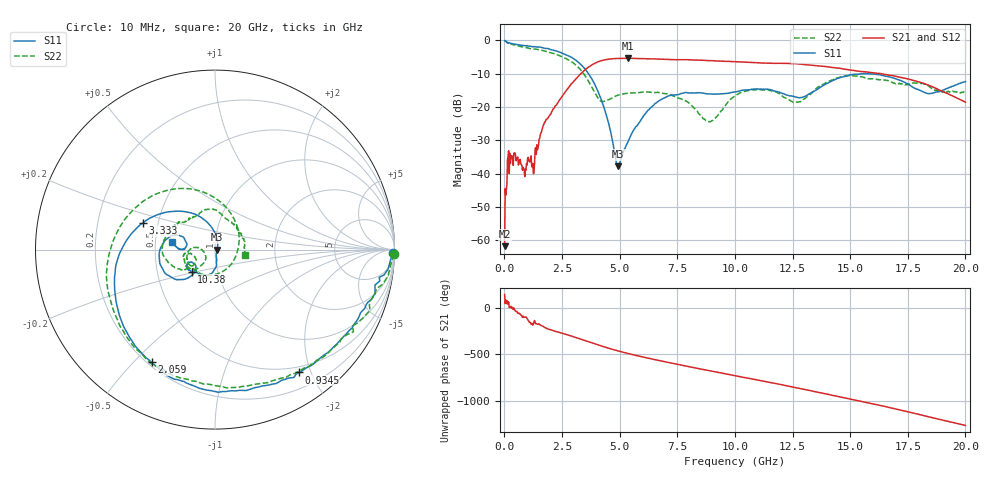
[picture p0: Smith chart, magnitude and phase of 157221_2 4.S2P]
!  2-Port S-parameters saved by WinCal
! VAR MeasName=S-Parameters (CALIBRATED_DATA) read from VNA (N5242A)
! VAR MeasDate=2015-5-26 16:47:30
! VAR NAME=157221_2 4
! VAR FILENAME=157221_2 4.S2P
! VAR DATE=2015-5-26 16:47:30
! VAR PHYS_PORTS=1,2
# Hz S DB R 50
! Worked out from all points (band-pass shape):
!   801 points, 10 MHz to 20 GHz, reference 50 ohm
!   highest |S21| = -5.38 dB at 5.357 GHz (marker M1); lowest = -61.8 dB at 10 MHz (marker M2)
!   |S21| within 3 dB of the highest: 3.582 GHz to 14.55 GHz (10.97 GHz wide, 121 % of centre)
!   lowest |S11| = -37.8 dB at 4.933 GHz (marker M3), VSWR 1.03, Z = 51.3 - j0.107 ohm
!   |S11| at or under -10 dB: 3.647 GHz to 15.52 GHz (11.88 GHz wide, 124 % of centre); 15.64509 GHz to 15.69706 GHz (51.97 MHz wide, 0.332 % of centre); 15.71 GHz to end of sweep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
!   |S22| runs from -24.4 to 0.0 dB; largest |S21 - S12| = 0.0096
!   S11 on the Smith chart (normalised r, x): 10 MHz: 35, -81; 934.5 MHz: 0.42, -1.82; 2.059 GHz: 0.22, -0.56; 3.333 GHz: 0.41, +0.15; 10.38 GHz: 0.75, -0.19; 20 GHz: 0.61, +0.05
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1e7  -0.08 -1.2  -61.78 139.9  -62.25 128.3  -0.03 -1.5
1.349375e8  -0.59 -10.7  -35.82 69.4  -35.91 67.2  -0.68 -15.7
2.348875e8  -0.77 -17.6  -33.91 4.3  -33.90 2.8  -0.85 -25.1
9.345375e8  -1.63 -55.7  -39.00 -101.2  -38.95 -101.1  -2.19 -78.9
1.284362e9  -1.93 -74.7  -39.74 -154.6  -39.71 -154.8  -2.63 -103.0
2.058975e9  -2.84 -119.4  -21.37 117.8  -21.36 117.7  -3.82 -155.3
3.333338e9  -7.36 159.6  -9.89 20.8  -9.87 20.4  -9.06 108.7
3.358325e9  -7.53 157.8  -9.72 18.7  -9.70 18.4  -9.27 106.4
4.2079e9  -17.88 99.0  -6.09 -52.1  -6.11 -52.3  -18.30 -17.6
4.932538e9  -37.85 -4.7  -5.43 -105.4  -5.42 -105.6  -16.48 -109.3
5.357325e9  -30.49 -78.4  -5.38 -132.6  -5.39 -132.8  -15.88 -133.1
6.681662e9  -18.28 -94.3  -5.61 152.9  -5.60 152.8  -15.68 -162.6
8.130938e9  -15.77 -126.0  -5.89 79.6  -5.87 79.3  -19.64 173.1
8.930538e9  -16.11 -133.7  -6.09 40.3  -6.07 39.9  -24.44 -153.1
1.0005e10  -15.44 -133.4  -6.41 -11.3  -6.41 -11.9  -16.69 -133.2
1.037981e10  -14.92 -136.7  -6.51 -29.3  -6.53 -29.7  -15.41 -139.8
1.18041e10  -15.32 -154.2  -6.91 -97.3  -6.87 -98.1  -15.58 -172.7
1.335332e10  -15.56 -132.7  -7.48 -176.3  -7.44 -176.7  -15.75 -145.1
1.492754e10  -10.54 -151.3  -8.82 101.9  -8.78 101.7  -10.64 -179.2
1.667666e10  -10.94 170.0  -10.43 8.6  -10.43 8.4  -12.22 141.9
1.810095e10  -15.27 163.4  -12.71 -74.2  -12.70 -75.1  -12.96 93.4
2e10  -12.37 170.4  -18.56 174.3  -18.59 172.9  -15.50 -10.8
